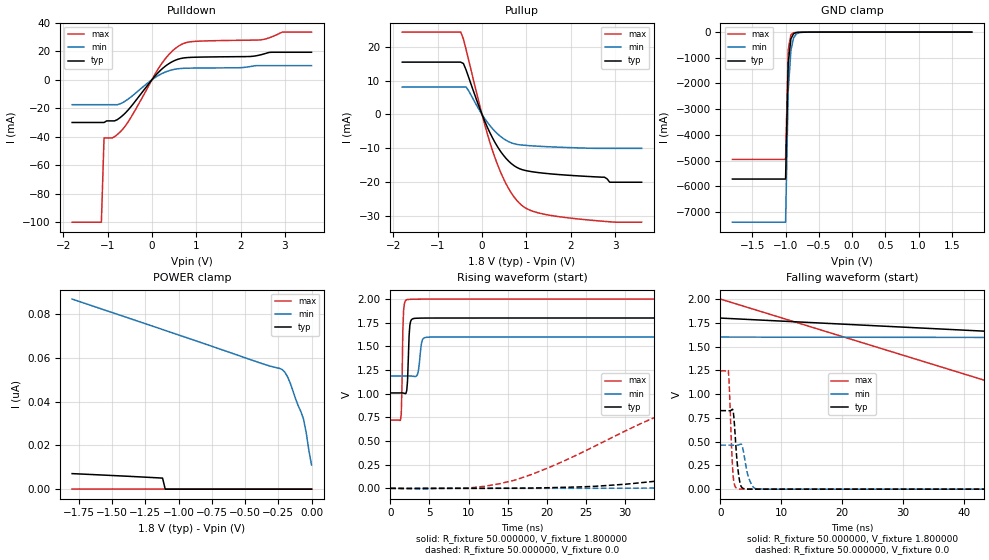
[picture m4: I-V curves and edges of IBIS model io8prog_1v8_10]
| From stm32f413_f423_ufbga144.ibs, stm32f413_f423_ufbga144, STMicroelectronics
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|   Model io8prog_1v8_10
[Model]  io8prog_1v8_10
Model_type I/O
Polarity   Non-Inverting
Enable   Active-Low
Vinl =   0.540000V
Vinh =   1.260000V
Vmeas =  0.900000V
Cref =   100.000000pF
Rref =   1.000000k
Vref =   1.800000V
C_comp   2.595400pF   2.437600pF   2.808600pF
[Temperature Range]   25.000000   0.125000k   -40.000000
[Pullup Reference]   1.800000V   1.600000V   2.000000V
[Pulldown Reference]   0.0V   0.0V   0.0V
[POWER Clamp Reference]   1.800000V   1.600000V   2.000000V
[GND Clamp Reference]   0.0V   0.0V   0.0V
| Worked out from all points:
|   slope of the pulldown table from 0 to 0.27 V, typ, clamps not added: 31 ohm
|   slope of the pullup table from 0 to 0.27 V, typ, clamps not added: 34.9 ohm
|   GND clamp passes 1 mA (typ) near -0.57 V on its own axis
|   rising waveform, R_fixture 50.000000, V_fixture 1.800000: 20-80 % time 213ps typ, 327ps min, 178ps max; typ from 1.01 V to 1.8 V
|   rising waveform, R_fixture 50.000000, V_fixture 0.0: 20-80 % time 42.7ns typ, 83.8ns min, 21ns max; typ from 0 V to 0.826 V
|   falling waveform, R_fixture 50.000000, V_fixture 1.800000: 20-80 % time 46.7ns typ, 84ns min, 43.8ns max; typ from 1.8 V to 1.01 V
|   falling waveform, R_fixture 50.000000, V_fixture 0.0: 20-80 % time 641ps typ, 956ps min, 471ps max; typ from 0.826 V to 0 V
[Pulldown]
|Voltage   I(typ)   I(min)   I(max)
-1.8V     -30mA      -17.52mA   -100mA
-1.14V    -30mA      -17.52mA   -100mA
-1.08V    -30mA      -17.52mA   -40.9mA
-840mV    -28.88mA   -17.52mA   -39.94mA
-600mV    -23.35mA   -14.94mA   -32.45mA
180mV     6.236mA    3.598mA    9.492mA
540mV     13.85mA    7.499mA    22.29mA
720mV     15.32mA    8.029mA    25.55mA
900mV     15.74mA    8.167mA    26.76mA
2.46V     17.56mA    9.912mA    28.02mA
2.94V     19.29mA    9.912mA    33.46mA
3.6V      19.29mA    9.912mA    33.46mA
[Pullup]
|Voltage   I(typ)   I(min)   I(max)
-1.8V     15.46mA    8.103mA    24.33mA
-480mV    15.46mA    8.103mA    24.33mA
-360mV    13.15mA    8.103mA    19.18mA
60mV      -1.95mA    -1.198mA   -2.977mA
300mV     -8.441mA   -5.092mA   -13.07mA
600mV     -13.78mA   -8.025mA   -21.88mA
900mV     -16.27mA   -9.02mA    -26.86mA
1.2V      -17.03mA   -9.318mA   -28.8mA
1.74V     -17.75mA   -9.658mA   -30.18mA
2.76V     -18.51mA   -10mA      -31.55mA
2.88V     -20mA      -10mA      -31.68mA
3.6V      -20mA      -10mA      -31.8mA
[GND_clamp]
|Voltage   I(typ)   I(min)   I(max)
-1.8V     -5.722A    -7.401A    -4.956A
-1V       -5.722A    -7.401A    -4.956A
-960mV    -1.203A    -2.294A    -680.3mA
-920mV    -260.8mA   -717.4mA   -103.7mA
-880mV    -62.26mA   -228.9mA   -23.84mA
-840mV    -19.05mA   -76.32mA   -11.31mA
-760mV    -5.573mA   -11.66mA   -6.2mA
-640mV    -2.048mA   -2.413mA   -2.197mA
1.8V      0A         0A         0A
[POWER_clamp]
|Voltage   I(typ)   I(min)   I(max)
-1.8V     7.116nA    87.04nA    0A
-1.12V    5.066nA    73.1nA     0A
-1.1V     0A         72.68nA    0A
-220mV    0A         54.75nA    0A
-200mV    0A         53.5nA     0A
-180mV    0A         51.44nA    0A
-160mV    0A         48.56nA    0A
-120mV    0A         41.39nA    0A
-60mV     0A         32.03nA    0A
-40mV     0A         25.87nA    0A
-20mV     0A         17.74nA    0A
0V        0A         11.07nA    0A
[Ramp]
| variable   typ   min   max
dV/dt_r  0.49566/42.66378n   0.27796/83.67398n   0.74712/20.99695n
dV/dt_f  0.47520/41.50240n   0.24780/72.61905n   0.76706/23.28960n
R_load = 50.000000
[Rising Waveform]
R_fixture= 50.000000
V_fixture= 1.800000
V_fixture_min= 1.600000
V_fixture_max= 2.000000
|time   V(typ)   V(min)   V(max)
0s        1.008V     1.187V     721.6mV
1.301ns   1.008V     1.187V     719.1mV
1.401ns   1.008V     1.187V     779.7mV
1.602ns   1.008V     1.187V     1.664V
1.702ns   1.006V     1.187V     1.879V
2.102ns   1.034V     1.187V     1.992V
2.503ns   1.724V     1.187V     1.997V
3.003ns   1.794V     1.183V     1.998V
4.605ns   1.799V     1.596V     1.999V
49.85ns   1.8V       1.6V       2V
[Rising Waveform]
R_fixture= 50.000000
V_fixture= 0.0
V_fixture_min= 0.0
V_fixture_max= 0.0
|time   V(typ)   V(min)   V(max)
0s        3.541nV    238.4nV    1.408nV
10.01ns   -100.7uV   -45.08uV   3.671mV
16.02ns   1.898mV    -32.52uV   89.43mV
36.04ns   96.74mV    3.52mV     826.4mV
46.05ns   223.2mV    10.06mV    1.07V
74.07ns   578.8mV    62.76mV    1.228V
116.1ns   783.6mV    224.6mV    1.244V
170.2ns   822mV      378mV      1.245V
228.2ns   825.6mV    438mV      1.245V
997ns     826.1mV    463.3mV    1.245V
[Falling Waveform]
R_fixture= 50.000000
V_fixture= 1.800000
V_fixture_min= 1.600000
V_fixture_max= 2.000000
|time   V(typ)   V(min)   V(max)
0s        1.8V       1.6V       2V
50.05ns   1.641V     1.596V     1.014V
100.1ns   1.13V      1.45V      741.6mV
150.2ns   1.033V     1.282V     723.9mV
200.2ns   1.014V     1.226V     722mV
250.2ns   1.01V      1.202V     721.6mV
400.4ns   1.008V     1.188V     721.6mV
4.955us   1.008V     1.187V     721.6mV
[Falling Waveform]
R_fixture= 50.000000
V_fixture= 0.0
V_fixture_min= 0.0
V_fixture_max= 0.0
|time   V(typ)   V(min)   V(max)
0s        826.1mV    463.3mV    1.245V
1.301ns   825.5mV    463.3mV    1.248V
1.401ns   825.2mV    463.3mV    1.169V
1.902ns   837.7mV    463.2mV    347.8mV
2.102ns   820.2mV    462.9mV    133.5mV
2.703ns   315.7mV    462.9mV    7.385mV
3.403ns   28.59mV    473.6mV    960.4uV
4.605ns   811.9uV    128mV      378.7uV
6.006ns   189.2uV    3.65mV     207.4uV
49.85ns   3.541nV    238.4nV    1.408nV
